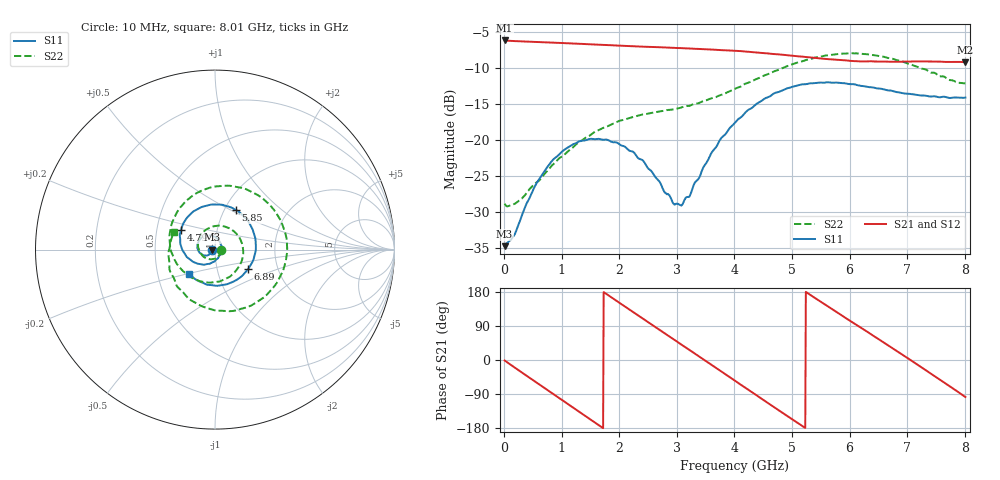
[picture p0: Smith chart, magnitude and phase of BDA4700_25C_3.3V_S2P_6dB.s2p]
!Agilent Technologies,E5071B,MY42404982,A.09.10
!Date: Mon Oct 20 18:05:30 2025
!Data & Calibration Information:
!Freq	S11:SOLT2(ON)	S21:SOLT2(ON)	S12:SOLT2(ON)	S22:SOLT2(ON)
# Hz S RI R 50
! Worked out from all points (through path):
!   801 points, 10 MHz to 8.01 GHz, reference 50 ohm
!   highest |S21| = -6.11 dB at 10 MHz (marker M1); lowest = -9.1 dB at 8.01 GHz (marker M2)
!   group delay of S21, straight-line fit = 283 ps
!   lowest |S11| = -34.8 dB at 10 MHz (marker M3), VSWR 1.04, Z = 48.2 - j0.0975 ohm
!   |S11| at or under -10 dB: start of sweep to end of sweep
!   |S22| runs from -29.2 to -7.9 dB; largest |S21 - S12| = 0.006
!   S11 on the Smith chart (normalised r, x): 10 MHz: 0.96, -0.00; 4.79 GHz: 0.67, +0.15; 5.85 GHz: 1.13, +0.53; 6.89 GHz: 1.41, -0.32; 8.01 GHz: 0.72, -0.20
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1e7  -0.0182 -0.00101  0.4946 -0.0106  0.4944 -0.0112  0.0359 -0.00289
1.7e8  -0.019 -0.0101  0.4652 -0.1542  0.4649 -0.1539  0.0313 -0.0173
3.3e8  -0.024 -0.0201  0.3983 -0.2806  0.3977 -0.2807  0.0224 -0.033
7.1e8  -0.0515 -0.0335  0.1243 -0.4639  0.1244 -0.4641  -0.0229 -0.054
1.02e9  -0.0811 -0.0218  -0.1409 -0.453  -0.141 -0.4532  -0.0702 -0.0331
1.35e9  -0.0984 0.0115  -0.3671 -0.291  -0.3668 -0.2912  -0.0943 0.0316
1.64e9  -0.0904 0.0473  -0.4577 -0.0679  -0.4575 -0.0679  -0.0675 0.0958
1.93e9  -0.0627 0.0735  -0.4251 0.1675  -0.4249 0.1676  0.00427 0.1318
2.32e9  -0.0124 0.0744  -0.2146 0.3949  -0.2144 0.395  0.1127 0.0956
2.68e9  0.026 0.0454  0.0648 0.4392  0.0639 0.4389  0.1574 -0.0136
3.08e9  0.0329 -0.0119  0.3328 0.2839  0.3296 0.286  0.098 -0.1375
3.53e9  -0.0123 -0.07  0.4273 -0.0404  0.4272 -0.0412  -0.0593 -0.1812
4.01e9  -0.1101 -0.0733  0.2417 -0.3424  0.2421 -0.3417  -0.2148 -0.0758
4.39e9  -0.1793 -0.00707  -0.0269 -0.4069  -0.0269 -0.4078  -0.2528 0.0869
4.79e9  -0.1893 0.1087  -0.2787 -0.2799  -0.277 -0.2817  -0.1684 0.2631
5.35e9  -0.0632 0.2406  -0.3682 0.0746  -0.3685 0.0723  0.1238 0.348
5.85e9  0.1148 0.2215  -0.1754 0.316  -0.1743 0.3157  0.3631 0.1669
6.25e9  0.21 0.1115  0.0594 0.3481  0.0653 0.3467  0.3886 -0.0863
6.68e9  0.2175 -0.0432  0.2792 0.2141  0.28 0.2134  0.2252 -0.2975
6.89e9  0.1839 -0.1091  0.3366 0.1013  0.3372 0.0994  0.1009 -0.3417
7.47e9  0.0134 -0.2016  0.2616 -0.2363  0.2612 -0.2369  -0.2106 -0.2061
8.01e9  -0.1446 -0.1348  -0.0472 -0.3459  -0.0462 -0.3464  -0.2276 0.0991
